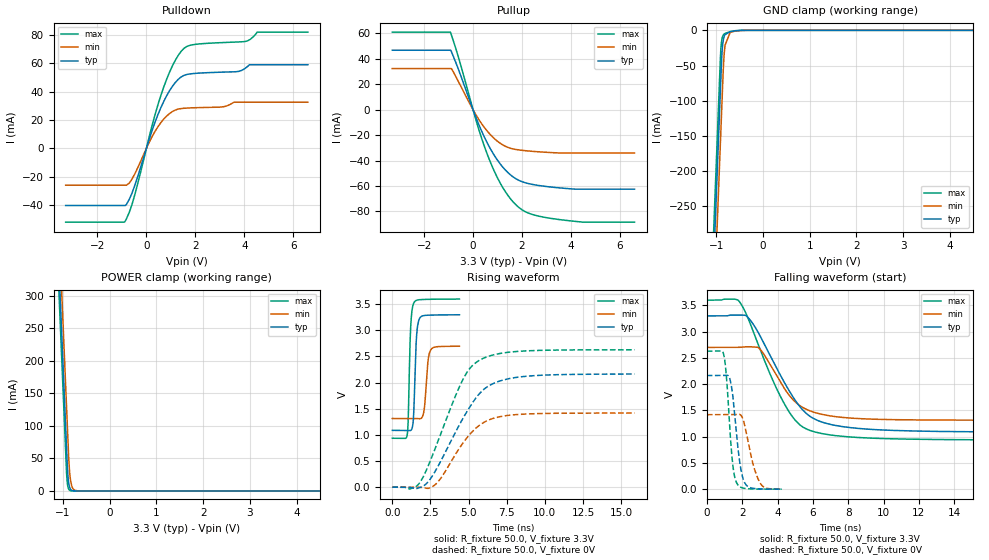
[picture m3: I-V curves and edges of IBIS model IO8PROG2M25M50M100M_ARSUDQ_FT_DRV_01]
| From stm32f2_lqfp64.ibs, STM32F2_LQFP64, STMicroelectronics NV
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| *** New cell (Generated with 5.14beta1 (Sep 20 2010 13:23:23))
[Model]   IO8PROG2M25M50M100M_ARSUDQ_FT_DRV_01
Model_type 3-state
Polarity   Non-Inverting
Enable   Active-Low
| CAP_THRESHOLD on pad IOV33 is "CMOS" :
| Rising=10.0% of vddio   Falling=90.0% of vddio
| C_comp min and max val. don't necessarily correlate with the min and max pvt
| but are the smallest and greatest pad capacitance found.
| var   typ   min   max
C_comp   2.14325pF  2.03775pF  2.26775pF
Vmeas = 1.65V   | Reference voltage for timing measurements
Cref  = 50.0pF   | Timing specification test load capacitance value
Rref  = 10.0MOhm   | Timing specification test load resistance value
Vref  = 1.65V   | Timing specification test load voltage
[Model Spec]
| variable   typ   min   max
[Temperature Range] 25.0 125.0 -40.0
| variable   typ   min   max
[Voltage Range] 3.3V 2.7V 3.6V
| variable   typ   min   max
[POWER Clamp Reference] 3.3V 2.7V 3.6V
| variable   typ   min   max
[GND Clamp Reference] 0V 0V 0V
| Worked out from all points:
|   slope of the pulldown table from 0 to 0.495 V, typ, clamps not added: 20 ohm
|   slope of the pullup table from 0 to 0.495 V, typ, clamps not added: 21.7 ohm
|   GND clamp passes 1 mA (typ) near -0.62 V on its own axis
|   POWER clamp passes 1 mA (typ) near -0.81 V on its own axis
|   rising waveform, R_fixture 50.0, V_fixture 3.3V: 20-80 % time 162ps typ, 213ps min, 146ps max; typ from 1.09 V to 3.3 V
|   falling waveform, R_fixture 50.0, V_fixture 3.3V: 20-80 % time 2.26ns typ, 1.77ns min, 2.11ns max; typ from 3.3 V to 1.09 V
|   rising waveform, R_fixture 50.0, V_fixture 0V: 20-80 % time 2.49ns typ, 2.07ns min, 2.19ns max; typ from 0 V to 2.17 V
|   falling waveform, R_fixture 50.0, V_fixture 0V: 20-80 % time 416ps typ, 599ps min, 330ps max; typ from 2.17 V to 0.001 V
[POWER Clamp]
-3.3V     4.11A      4.173A     4.072A
-1.09V    352.5mA    415.9mA    314.5mA
-1.05V    284.5mA    347.9mA    246.5mA
-1.01V    216.5mA    279.9mA    178.5mA
-920mV    63.51mA    126.9mA    25.85mA
-900mV    31.51mA    92.9mA     9.552mA
-890mV    21.35mA    75.9mA     5.807mA
-870mV    9.804mA    44.01mA    2.146mA
-840mV    3.05mA     18.36mA    482.1uA
-780mV    295.2uA    3.194mA    24.34uA
-660mV    2.764uA    96.54uA    62.42nA
6.6V      0A         0A         0A
[GND Clamp]
-3.3V     -4.149A    -4.223A    -4.103A
-1.06V    -340.6mA   -415.4mA   -294.5mA
-940mV    -136.6mA   -211.4mA   -90.54mA
-910mV    -85.55mA   -160.4mA   -39.54mA
-900mV    -68.55mA   -143.4mA   -26.55mA
-880mV    -36.73mA   -109.4mA   -13.46mA
-860mV    -19.54mA   -75.4mA    -8.234mA
-840mV    -11.29mA   -44.89mA   -5.954mA
-810mV    -6.008mA   -21.13mA   -4.401mA
-700mV    -1.958mA   -2.906mA   -1.882mA
-470mV    -105.5uA   -263.9uA   -47.31uA
6.6V      9.456nA    1.185uA    63.86pA
| variable   typ   min   max
[Pullup Reference] 3.3V 2.7V 3.6V
| variable   typ   min   max
[Pulldown Reference] 0V 0V 0V
[Pullup]
-3.3V     46.81mA    32.38mA    61.09mA
-930mV    46.81mA    32.38mA    61.09mA
-880mV    45.47mA    32.38mA    58.55mA
-590mV    31.39mA    21.85mA    40.84mA
240mV     -11.89mA   -7.822mA   -15.87mA
590mV     -26.5mA    -17.07mA   -35.52mA
1.18V     -44.36mA   -27.27mA   -60.11mA
1.54V     -51.43mA   -30.39mA   -70.35mA
1.89V     -55.75mA   -31.69mA   -77.18mA
2.48V     -58.98mA   -32.83mA   -82.75mA
3.6V      -61.62mA   -34.07mA   -86.61mA
6.6V      -62.54mA   -34.07mA   -88.51mA
[Pulldown]
-3.3V     -40.26mA   -25.94mA   -51.99mA
-870mV    -40.25mA   -25.94mA   -51.33mA
-700mV    -35.92mA   -24.51mA   -45.06mA
-470mV    -25.89mA   -17.87mA   -32.39mA
240mV     12.97mA    8.52mA     16.62mA
590mV     28.62mA    18.11mA    37.2mA
1.07V     43.85mA    26mA       58.31mA
1.54V     51.42mA    28.24mA    70.48mA
2.01V     52.82mA    28.63mA    73.27mA
4.01V     56.01mA    32.56mA    75.18mA
4.53V     58.89mA    32.56mA    81.88mA
6.6V      58.89mA    32.56mA    81.88mA
[Ramp]
dV/dt_r 1.29886V/2.48978ns 851.30661mV/2.07003ns 1.57728V/2.18698ns
dV/dt_f 1.32782V/2.26478ns 831.60249mV/1.76759ns 1.59819V/2.1086ns
R_load = 50.0
| Removed startup time: 0s 0s 0s  .
| Removed end time: 4.4ns.
[Rising Waveform]
R_fixture   = 50.0
V_fixture   = 3.3V
V_fixture_min = 2.7V
V_fixture_max = 3.6V
0s        1.087V     1.314V     936.3mV
982ps     1.087V     1.314V     1.009V
1.044ns   1.086V     1.314V     1.303V
1.206ns   1.086V     1.314V     3.067V
1.414ns   1.482V     1.314V     3.527V
1.577ns   2.83V      1.313V     3.574V
1.782ns   3.224V     1.309V     3.586V
2.079ns   3.283V     1.462V     3.591V
2.505ns   3.292V     2.619V     3.594V
4.402ns   3.298V     2.698V     3.598V
| Removed startup time: 0s 0s 0s  .
| Removed end time: 20.335ns.
[Falling Waveform]
R_fixture   = 50.0
V_fixture   = 3.3V
V_fixture_min = 2.7V
V_fixture_max = 3.6V
0s        3.3V       2.7V       3.6V
1.825ns   3.315V     2.701V     3.579V
2.28ns    3.288V     2.711V     3.297V
2.95ns    2.958V     2.685V     2.719V
4.355ns   2.052V     1.936V     1.646V
5.14ns    1.627V     1.623V     1.264V
5.8ns     1.396V     1.496V     1.123V
7.035ns   1.23V      1.393V     1.031V
9.28ns    1.139V     1.335V     972.6mV
20.35ns   1.087V     1.314V     936.6mV
| Removed startup time: 0s 0s 0s  .
| Removed end time: 15.87ns.
[Rising Waveform]
R_fixture   = 50.0
V_fixture   = 0V
V_fixture_min = 0V
V_fixture_max = 0V
0s        7.764nV    280.7nV    5.72nV
1.14ns    -487.6uV   -6.875uV   -37.26mV
1.835ns   -3.896mV   -1.798mV   101.5mV
2.89ns    344.2mV    69.88mV    799.6mV
4.515ns   1.256V     796.6mV    1.993V
5.1ns     1.543V     1.018V     2.279V
5.725ns   1.793V     1.187V     2.43V
6.775ns   2.003V     1.33V      2.541V
8.325ns   2.108V     1.392V     2.6V
15.88ns   2.165V     1.419V     2.629V
| Removed startup time: 0s 0s 0s  .
| Removed end time: 4.234ns.
[Falling Waveform]
R_fixture   = 50.0
V_fixture   = 0V
V_fixture_min = 0V
V_fixture_max = 0V
0s        2.165V     1.419V     2.629V
961ps     2.166V     1.419V     2.554V
1.14ns    2.171V     1.419V     2.024V
1.351ns   2.034V     1.418V     910.6mV
1.515ns   1.629V     1.42V      345mV
1.702ns   962mV      1.424V     111.2mV
1.964ns   314.6mV    1.393V     29.86mV
2.245ns   73.62mV    1.056V     11.04mV
3.029ns   4.627mV    110.5mV    1.903mV
4.236ns   781.4uV    1.128mV    585.5uV
